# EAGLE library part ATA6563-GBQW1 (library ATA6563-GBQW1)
CAN Interface IC CAN TRX with VIO PIN (DFN8) Source: Datasheet
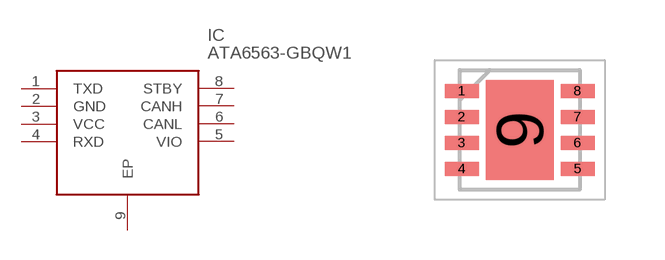
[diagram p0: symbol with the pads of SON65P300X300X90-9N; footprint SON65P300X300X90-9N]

Designator prefix IC

## ATA6563-GBQW1 (Description: CAN Interface IC CAN TRX with VIO PIN (DFN8); Height: 0.9mm; Manufacturer_Name: Microchip; Manufacturer_Part_Number: ATA6563-GBQW1; Mouser_Part_Number: 579-ATA6563-GBQW1; Mouser_Price-Stock: https://www.mouser.co.uk/ProductDetail/Microchip-Technology/ATA6563-GBQW1?qs=byeeYqUIh0OFDnqHLfeuvg%3D%3D)  [SON65P300X300X90-9N]
1  TXD
2  GND
3  VCC
4  RXD
5  VIO
6  CANL
7  CANH
8  STBY
9  EP

## Footprint SON65P300X300X90-9N (pad centres in mm)
3x3 mm Body [VDFN]
smd 0.85 x 0.35: 1 -1.45,0.975; 2 -1.45,0.325; 3 -1.45,-0.325; 4 -1.45,-0.975; 5 1.45,-0.975; 6 1.45,-0.325; 7 1.45,0.325; 8 1.45,0.975
smd 1.7 x 2.5: 9 0,0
